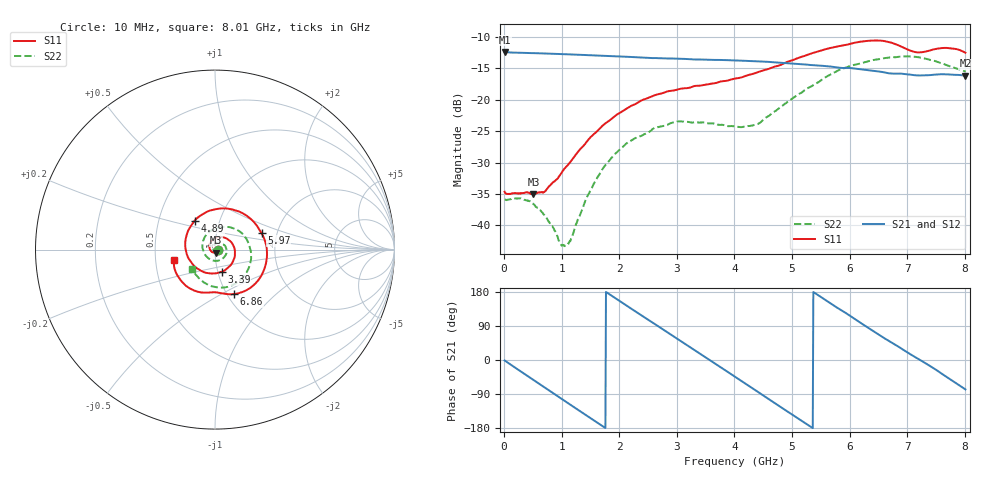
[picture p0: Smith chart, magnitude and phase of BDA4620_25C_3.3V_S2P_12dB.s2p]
!Agilent Technologies,E5071B,MY42404982,A.09.10
!Date: Wed May 06 08:51:02 2026
!Data & Calibration Information:
!Freq	S11:SOLT2(ON)	S21:SOLT2(ON)	S12:SOLT2(ON)	S22:SOLT2(ON)
# Hz S RI R 50
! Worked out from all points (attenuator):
!   801 points, 10 MHz to 8.01 GHz, reference 50 ohm
!   highest |S21| = -12.43 dB at 10 MHz (marker M1); lowest = -16.2 dB at 8.01 GHz (marker M2)
!   lowest |S11| = -35.1 dB at 510 MHz (marker M3), VSWR 1.04, Z = 50.4 - j1.73 ohm
!   |S11| at or under -10 dB: start of sweep to end of sweep
!   |S22| runs from -43.3 to -13.1 dB; largest |S21 - S12| = 0.001
!   S11 on the Smith chart (normalised r, x): 10 MHz: 1.04, -0.00; 3.39 GHz: 1.04, -0.26; 4.89 GHz: 0.76, +0.26; 5.97 GHz: 1.66, +0.33; 6.86 GHz: 1.07, -0.57; 8.01 GHz: 0.62, -0.07
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1e7  0.0185 -0.00139  0.2391 -0.0052  0.2393 -0.00512  0.016 -0.000709
5.1e8  0.00383 -0.0172  0.1422 -0.1865  0.1424 -0.187  0.012 -0.00859
7.1e8  -0.00844 -0.0166  0.0677 -0.2231  0.0675 -0.2235  0.00618 -0.0102
1.04e9  -0.0279 -0.000545  -0.0662 -0.2204  -0.0665 -0.2207  -0.00501 -0.00483
1.16e9  -0.0307 0.0099  -0.1107 -0.2005  -0.1111 -0.2007  -0.00775 -0.000225
1.35e9  -0.0302 0.0287  -0.1694 -0.1515  -0.1695 -0.1517  -0.00989 0.00861
1.59e9  -0.0164 0.0521  -0.2143 -0.068  -0.2146 -0.0682  -0.00718 0.0215
1.9e9  0.0199 0.0698  -0.2156 0.052  -0.2158 0.0522  0.00711 0.0351
2.31e9  0.0778 0.0525  -0.1255 0.1775  -0.1256 0.1778  0.0363 0.035
2.68e9  0.1107 -0.00333  0.00493 0.2138  0.00523 0.2141  0.0581 0.0167
3.39e9  0.0367 -0.1239  0.1986 0.0647  0.1991 0.0645  0.0456 -0.0473
4.01e9  -0.1127 -0.0945  0.1472 -0.1431  0.1473 -0.1434  -0.0279 -0.0547
4.41e9  -0.1653 0.013  0.0198 -0.2003  0.0196 -0.2009  -0.0636 -0.00841
4.89e9  -0.1127 0.162  -0.1332 -0.1435  -0.1332 -0.1439  -0.0512 0.0781
5.35e9  0.0466 0.2299  -0.1883 -0.00418  -0.1886 -0.00418  0.033 0.1245
5.97e9  0.2591 0.0923  -0.0903 0.1548  -0.0903 0.155  0.17 0.067
6.33e9  0.2842 -0.0764  0.0172 0.1707  0.0174 0.1708  0.2011 -0.0237
6.68e9  0.1837 -0.2216  0.1032 0.125  0.1035 0.1254  0.1787 -0.1211
6.86e9  0.1047 -0.2479  0.1338 0.0903  0.1342 0.0905  0.1475 -0.1629
7.18e9  0.00324 -0.2376  0.1556 0.0105  0.1559 0.0106  0.0604 -0.2097
7.54e9  -0.1135 -0.2286  0.138 -0.0794  0.1381 -0.0793  -0.0412 -0.1945
8.01e9  -0.2297 -0.0565  0.0334 -0.1514  0.0338 -0.1518  -0.1285 -0.1065
